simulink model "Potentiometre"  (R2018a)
settings: Solver=FixedStepAuto  StartTime=0.0  StopTime=inf  RelTol=1e-3  EnableMultiTasking=on
libraries: arduinolib x1

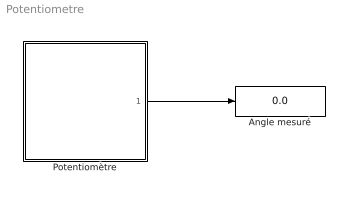
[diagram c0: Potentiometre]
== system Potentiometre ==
  Angle mesuré : Display
  Potentiomètre : Subsystem
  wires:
  Potentiomètre/1(Out1) -> Angle mesuré/1

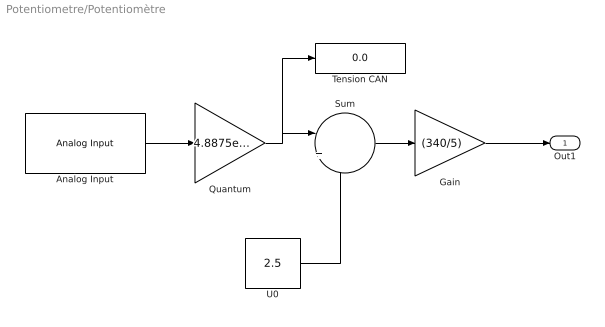
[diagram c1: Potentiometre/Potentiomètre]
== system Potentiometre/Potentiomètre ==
  Analog Input : arduinolib/Analog Input  pinNumber=5  ReadResultsOnly=off  ConversionTriggerSource=Software  ExternalTriggerType=uint32(0)  OutputDataType=uint16  EnableConversionCompleteNotify=off  EnableOuputStatus=off  SampleTime=0.01  blockPlatform=arduino
  Gain : Gain  Gain=(340/5)
  Quantum : Gain  Gain=4.8875e-3
  Sum : Sum  Inputs=|+-
  Tension CAN : Display
  U0 : Constant  Value=2.5
  Out1 : Outport
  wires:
  Gain/1 -> Out1/1
  Analog Input/1 -> Quantum/1
  Quantum/1 -> Tension CAN/1, Sum/1
  U0/1 -> Sum/2
  Sum/1 -> Gain/1
